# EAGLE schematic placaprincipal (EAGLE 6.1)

## Sheet 1 of 3: Diagrama Esquematico de Microcontrolador ATMEGA32U4: El siguiente esquema muestra las distribucion de los pines del microcontrolador junto con el Puerto USB que contiene este, ademas se tiene que tomar en cuenta que el se tiene 2 fuentes distintas la cual es una diferente del otra ya que una es VCC1 alimentacion del todo el circuito y VCC2 que es la alimentacion que viene del puerto USB
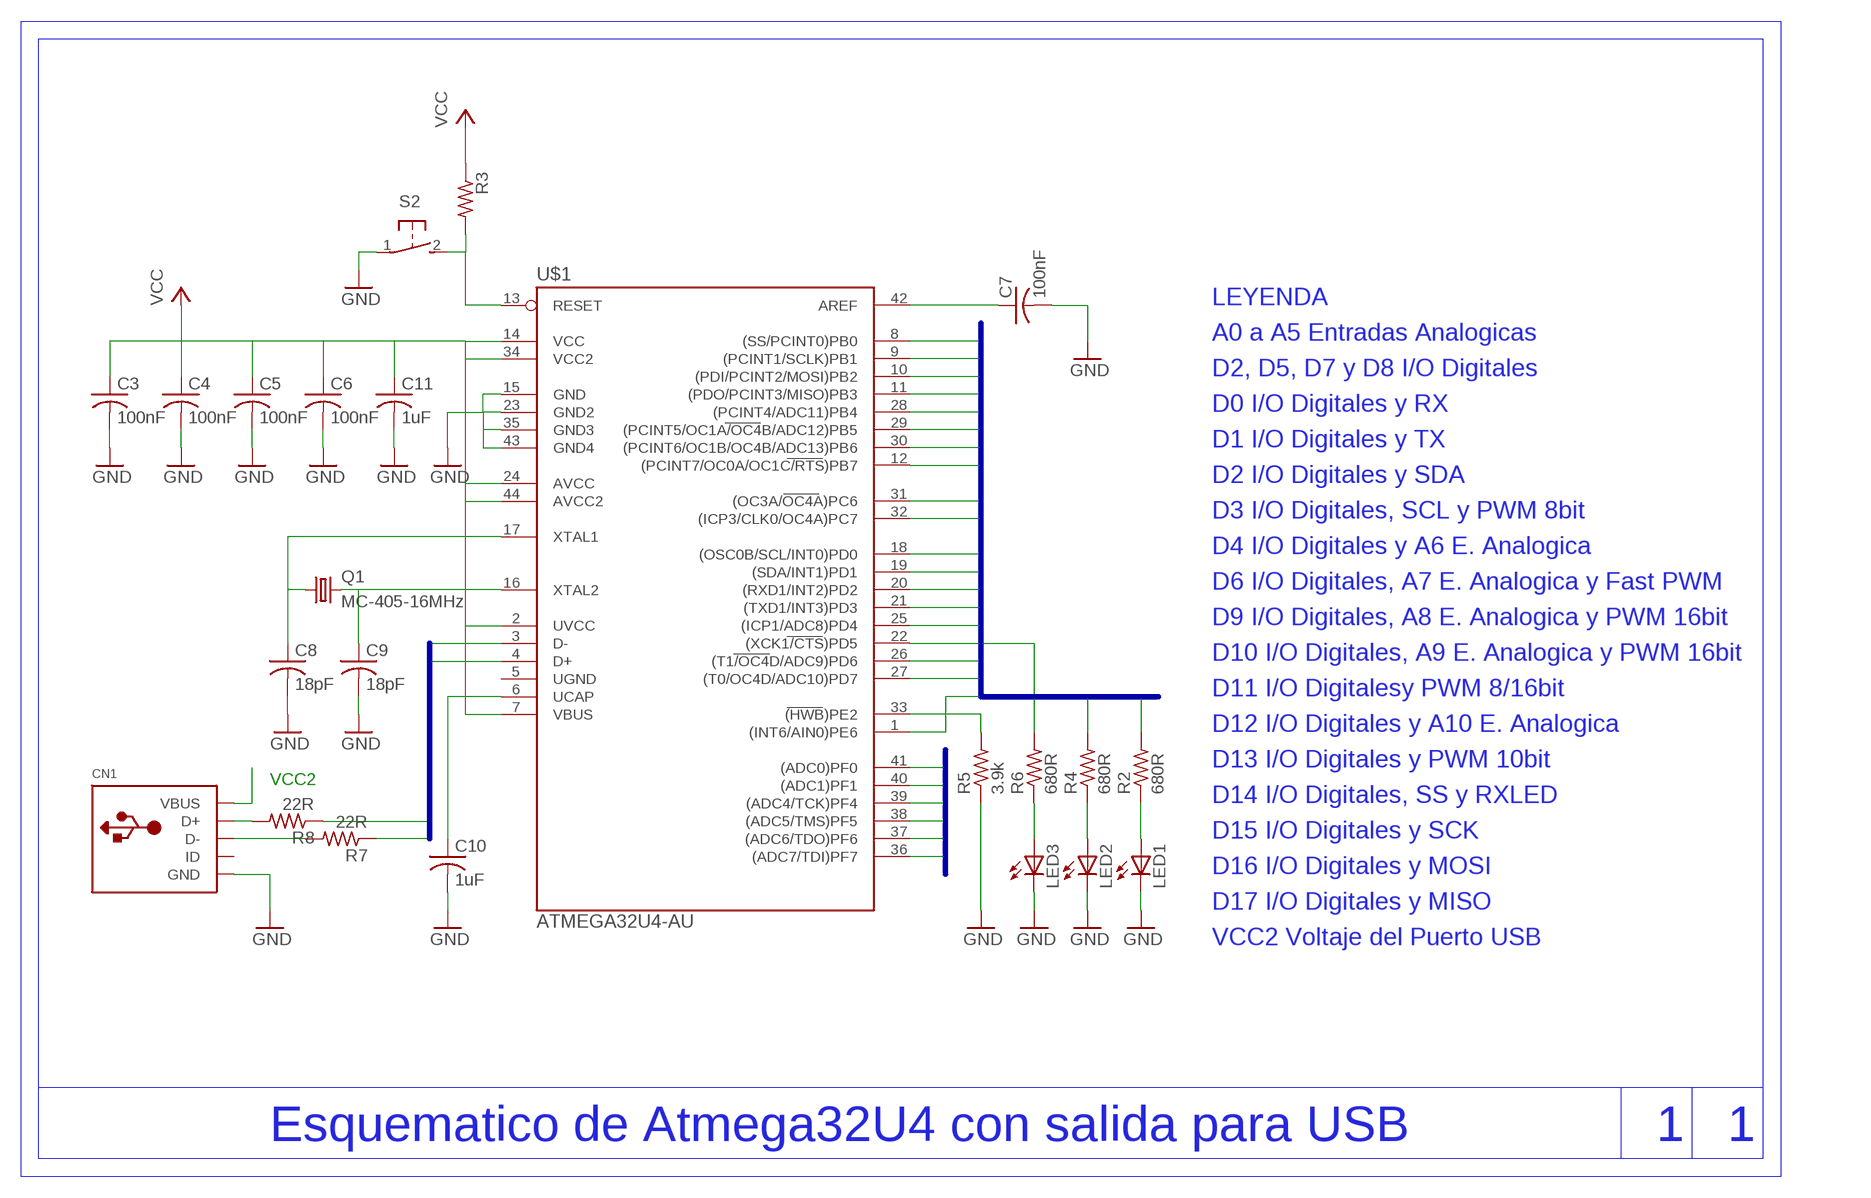
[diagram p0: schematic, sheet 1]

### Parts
C3  100nF  C-USC1206  [C1206]
C4  100nF  C-USC1206  [C1206]
C5  100nF  C-USC1206  [C1206]
C6  100nF  C-USC1206  [C1206]
C7  100nF  C-USC1206  [C1206]
C8  18pF  C-USC1206  [C1206]
C9  18pF  C-USC1206  [C1206]
C10  1uF  C-USC1206  [C1206]
C11  1uF  C-USC1206  [C1206]
CN1  USBMINIB  [USB-MINIB]
LED1  LEDSMT1206  [1206]
LED2  LEDSMT1206  [1206]
LED3  LEDSMT1206  [1206]
Q1  MC-405-16MHz  MC-405  [MC-405]
R2  680R  R-US_R1206  [R1206]
R3  R-US_R1206  [R1206]
R4  680R  R-US_R1206  [R1206]
R5  3.9k  R-US_R1206  [R1206]
R6  680R  R-US_R1206  [R1206]
R7  22R  R-US_R1206  [R1206]
R8  22R  R-US_R1206  [R1206]
S2  31-XX  [B3F-31XX]
U$1  ATMEGA32U4-AU  [TQFP44]

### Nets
A0: U$1.36((ADC7/TDI)PF7)
A1: U$1.37((ADC6/TDO)PF6)
A2: U$1.38((ADC5/TMS)PF5)
A3: U$1.39((ADC4/TCK)PF4)
A4: U$1.40((ADC1)PF1)
A5: U$1.41((ADC0)PF0)
D0: U$1.20((RXD1/INT2)PD2)
D1: U$1.21((TXD1/INT3)PD3)
D2: U$1.19((SDA/INT1)PD1) ; also sheet 2
D3: U$1.18((OSC0B/SCL/INT0)PD0) ; also sheet 2
D4: U$1.25((ICP1/ADC8)PD4)
D5: U$1.31((OC3A/OC4A)PC6)
D6: U$1.27((T0/OC4D/ADC10)PD7)
D7: U$1.1((INT6/AIN0)PE6)
D8: U$1.28((PCINT4/ADC11)PB4) ; also sheet 2
D9: U$1.29((PCINT5/OC1A/OC4B/ADC12)PB5)
D10: U$1.30((PCINT6/OC1B/OC4B/ADC13)PB6) ; also sheet 2
D11: U$1.12((PCINT7/OC0A/OC1C/RTS)PB7) ; also sheet 2
D12: U$1.26((T1/OC4D/ADC9)PD6) ; also sheet 2
D13: R4.2 U$1.32((ICP3/CLK0/OC4A)PC7) ; also sheet 2
D14: R2.2 U$1.8((SS/PCINT0)PB0)
D15: U$1.9((PCINT1/SCLK)PB1) ; also sheet 2
D16: U$1.10((PDI/PCINT2/MOSI)PB2) ; also sheet 2
D17: U$1.11((PDO/PCINT3/MISO)PB3) ; also sheet 2
DATA0: R7.1 U$1.3(D-)
DATA1: R8.1 U$1.4(D+)
GND: C3.2 C4.2 C5.2 C6.2 C7.2 C8.2 C9.2 C10.2 C11.2 CN1.GND LED1.C LED2.C LED3.C R5.1 S2.1(P) U$1.15(GND) U$1.23(GND2) U$1.35(GND3) U$1.43(GND4) ; also sheet 2,3
N$1: R5.2 U$1.33((HWB)PE2)
N$4: C10.1 U$1.6(UCAP)
N$5: C9.1 Q1.2 U$1.16(XTAL2)
N$6: C7.1 U$1.42(AREF)
N$7: C8.1 Q1.1 U$1.17(XTAL1)
N$9: R6.2 U$1.22((XCK1/CTS)PD5)
N$10: CN1.D- R7.2
N$11: R3.2 S2.2(S) U$1.13(RESET)
N$12: CN1.D+ R8.2
N$13: LED3.A R6.1
N$16: LED1.A R2.1
N$17: LED2.A R4.1
VCC: C3.1 C4.1 C5.1 C6.1 C11.1 R3.1 U$1.2(UVCC) U$1.7(VBUS) U$1.14(VCC) U$1.24(AVCC) U$1.34(VCC2) U$1.44(AVCC2) ; also sheet 2,3
VCC2: CN1.VBUS ; also sheet 3
Unconnected: CN1.ID U$1.5(UGND)

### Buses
A[0..5]
D[0..17]
DATA[0..1]

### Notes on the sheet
- LEYENDA
- A0 a A5 Entradas Analogicas
- D2, D5, D7 y D8 I/O Digitales
- D0 I/O Digitales y RX
- D1 I/O Digitales y TX
- D2 I/O Digitales y SDA
- D3 I/O Digitales, SCL y PWM 8bit
- D4 I/O Digitales y A6 E. Analogica
- D6 I/O Digitales, A7 E. Analogica y Fast PWM
- D9 I/O Digitales, A8 E. Analogica y PWM 16bit
- D10 I/O Digitales, A9 E. Analogica y PWM 16bit
- D11 I/O Digitalesy PWM 8/16bit
- D12 I/O Digitales y A10 E. Analogica
- D13 I/O Digitales y PWM 10bit
- VCC2
- D14 I/O Digitales, SS y RXLED
- D15 I/O Digitales y SCK
- D16 I/O Digitales y MOSI
- D17 I/O Digitales y MISO
- VCC2 Voltaje del Puerto USB
- Esquematico de Atmega32U4 con salida para USB | 1 | 1

## Sheet 2 of 3: Esquematicos de EPROM, RTC, SD y SIM908: Los cuales van unidos a la placa principal del microcontrolador mediante buses que nos permiten unir pines, en nuestro caso nos permite unir a las I/O digitales.
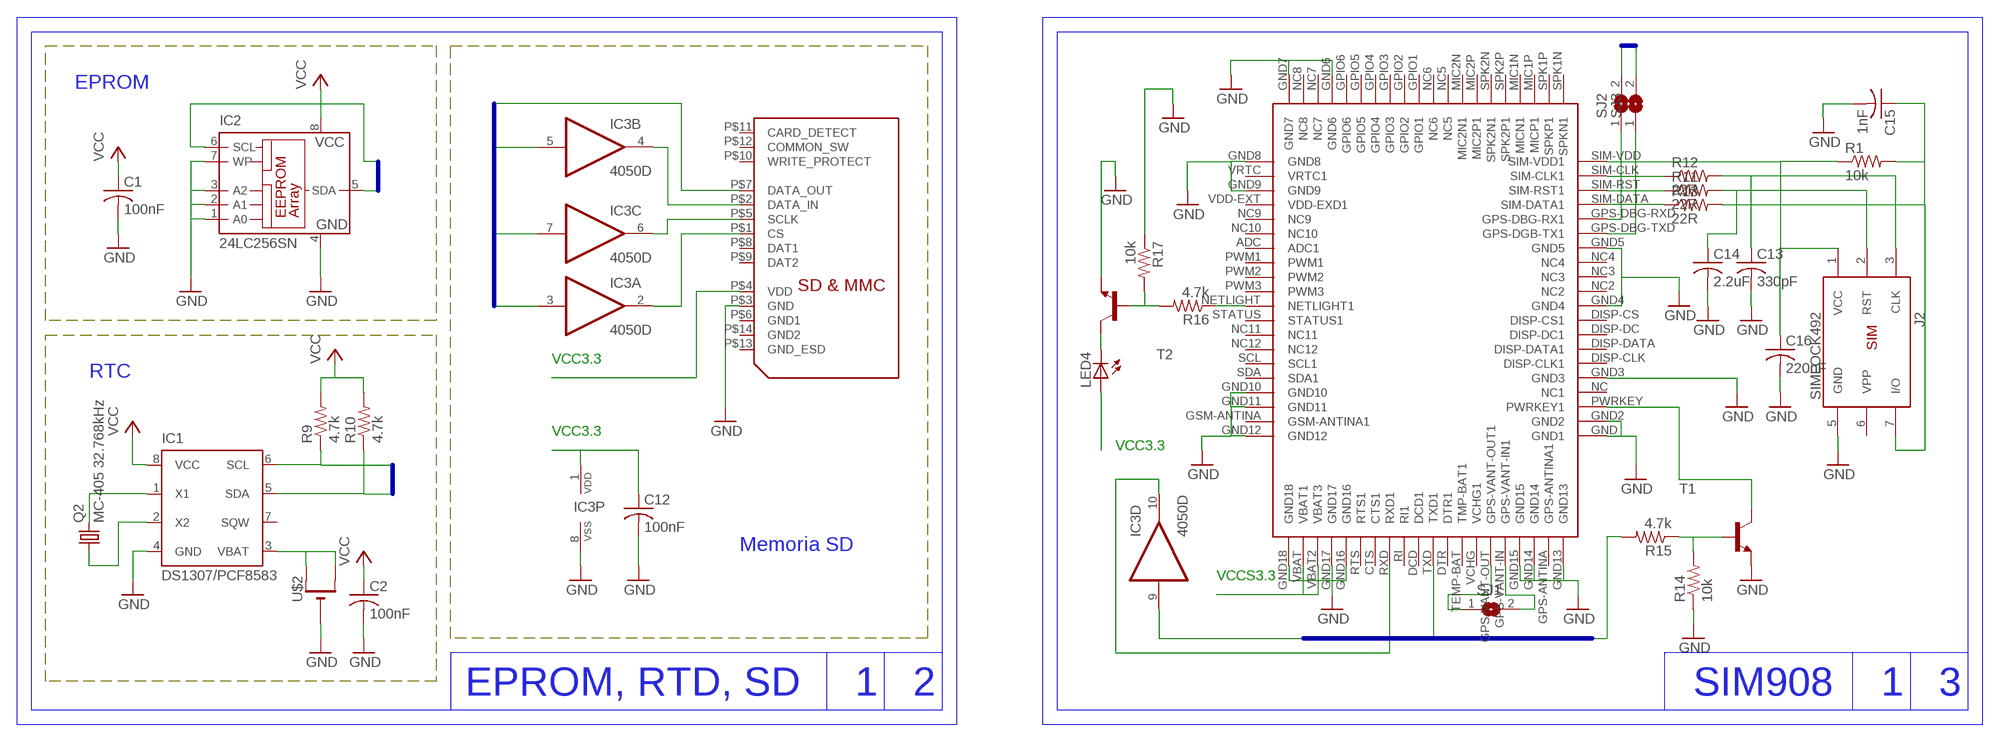
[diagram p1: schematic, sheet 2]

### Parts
C1  100nF  C-USC1206  [C1206]
C2  100nF  C-USC1206  [C1206]
C12  100nF  C-USC1206  [C1206]
C13  330pF  C-USC1206  [C1206]
C14  2.2uF  C-USC1206  [C1206]
C15  1nF  C-USC1206  [C1206]
C16  220nF  C-USC1206  [C1206]
IC1  DS1307/PCF8583  [SO8-7_5+SOIC8]
IC2  24LC256SN  [SO-08]
IC3  4050D  [SO16]
J2  SIMLOCK492  [5002]
LED4  LEDSMT1206  [1206]
Q2  MC-405 32.768kHz  MC-405  [MC-405]
R1  10k  R-US_R1206  [R1206]
R9  4.7k  R-US_R1206  [R1206]
R10  4.7k  R-US_R1206  [R1206]
R11  22R  R-US_R1206  [R1206]
R12  22R  R-US_R1206  [R1206]
R13  22R  R-US_R1206  [R1206]
R14  10k  R-US_R1206  [R1206]
R15  4.7k  R-US_R1206  [R1206]
R16  4.7k  R-US_R1206  [R1206]
R17  10k  R-US_R1206  [R1206]
SD1  FPS009-2405-0  [FPS009-2405]
SJ1  SJ  [SJ]
SJ2  SJ  [SJ]
SJ3  SJ  [SJ]
T1  BC817-16-NPN-SOT23-BEC  [SOT23-BEC]
T2  BC817-16-NPN-SOT23-BEC  [SOT23-BEC]
U$2  CR1220SMT  [CR1220-SMD]
U$4  SIM908  [SIM908]

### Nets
D2: IC1.5(SDA) IC2.5(SDA) R10.1 ; also sheet 1
D3: IC1.6(SCL) IC2.6(SCL) R9.1 ; also sheet 1
D8: R15.2 ; also sheet 1
D10: SJ2.2 ; also sheet 1
D11: IC3.3(A:I) SJ3.2 ; also sheet 1
D12: IC3.9(D:I) ; also sheet 1
D13: U$4.TXD(TXD1) ; also sheet 1
D15: IC3.7(C:I) ; also sheet 1
D16: IC3.5(B:I) ; also sheet 1
D17: SD1.P$7(DATA_OUT) ; also sheet 1
GND: C1.2 C2.2 C12.2 C13.2 C14.2 C15.2 C16.2 IC1.4(GND) IC2.1(A0) IC2.2(A1) IC2.3(A2) IC2.4(GND) IC2.7(WP) IC3.8(P:VSS) J2.5(GND) R14.1 R17.1 SD1.P$3(GND) T1.E T2.E U$2.- U$4.GND2 U$4.GND3 U$4.GND4 U$4.GND5 U$4.GND6 U$4.GND7 U$4.GND8 U$4.GND9 U$4.GND10 U$4.GND11 U$4.GND12 U$4.GND13 U$4.GND14 U$4.GND15 U$4.GND16 U$4.GND17 U$4.GND18 U$4.GND(GND1) ; also sheet 1,3
N$2: IC1.3(VBAT) U$2.+$1(+) U$2.+$2(+1)
N$3: IC1.1(X1) Q2.2
N$8: IC1.2(X2) Q2.1
N$14: IC3.2(A:O) SD1.P$1(CS)
N$15: IC3.4(B:O) SD1.P$2(DATA_IN)
N$18: IC3.6(C:O) SD1.P$5(SCLK)
N$19: C14.1 J2.2(RST) R11.2
N$20: C13.1 J2.3(CLK) R12.2
N$21: C15.1 J2.7(I/O) R1.2 R13.2
N$22: C16.1 J2.1(VCC) R1.1 U$4.SIM-VDD(SIM-VDD1)
N$23: R13.1 U$4.SIM-DATA(SIM-DATA1)
N$24: R12.1 U$4.SIM-CLK(SIM-CLK1)
N$25: R11.1 U$4.SIM-RST(SIM-RST1)
N$28: IC3.10(D:O) U$4.RXD(RXD1)
N$29: SJ2.1 U$4.GPS-DBG-RXD(GPS-DBG-RX1)
N$30: SJ3.1 U$4.GPS-DBG-TXD(GPS-DGB-TX1)
N$31: T1.C U$4.PWRKEY(PWRKEY1)
N$32: R14.2 R15.1 T1.B
N$33: R16.1 U$4.NETLIGHT(NETLIGHT1)
N$34: LED4.C T2.C
N$35: R16.2 R17.2 T2.B
N$38: SJ1.2 U$4.GPS-VANT-IN(GPS-VANT-IN1)
N$39: SJ1.1 U$4.GPS-VANT-OUT(GPS-VANT-OUT1)
VCC: C1.1 C2.1 IC1.8(VCC) IC2.8(VCC) R9.2 R10.2 ; also sheet 1,3
VCC3.3: C12.1 IC3.1(P:VDD) LED4.A SD1.P$4(VDD) U$4.VBAT2(VBAT3) U$4.VBAT(VBAT1) ; also sheet 3
Unconnected: IC1.7(SQW) IC3.11(E:I) IC3.12(E:O) IC3.14(F:I) IC3.15(F:O) J2.6(VPP) SD1.P$6(GND1) SD1.P$8(DAT1) SD1.P$9(DAT2) SD1.P$10(WRITE_PROTECT) SD1.P$11(CARD_DETECT) SD1.P$12(COMMON_SW) SD1.P$13(GND_ESD) SD1.P$14(GND2) U$4.ADC(ADC1) U$4.CTS(CTS1) U$4.DCD(DCD1) U$4.DISP-CLK(DISP-CLK1) U$4.DISP-CS(DISP-CS1) U$4.DISP-DATA(DISP-DATA1) U$4.DISP-DC(DISP-DC1) U$4.DTR(DTR1) U$4.GPIO1 U$4.GPIO2 U$4.GPIO3 U$4.GPIO4 U$4.GPIO5 U$4.GPIO6 U$4.GPS-ANTINA(GPS-ANTINA1) U$4.GSM-ANTINA(GSM-ANTINA1) U$4.MIC1N(MICN1) U$4.MIC1P(MICP1) U$4.MIC2N(MIC2N1) U$4.MIC2P(MIC2P1) U$4.NC2 U$4.NC3 U$4.NC4 U$4.NC5 U$4.NC6 U$4.NC7 U$4.NC8 U$4.NC9 U$4.NC10 U$4.NC11 U$4.NC12 U$4.NC(NC1) U$4.PWM1 U$4.PWM2 U$4.PWM3 U$4.RI(RI1) U$4.RTS(RTS1) U$4.SCL(SCL1) U$4.SDA(SDA1) U$4.SPK1N(SPKN1) U$4.SPK1P(SPKP1) U$4.SPK2N(SPK2N1) U$4.SPK2P(SPK2P1) U$4.STATUS(STATUS1) U$4.TEMP-BAT(TMP-BAT1) U$4.VCHG(VCHG1) U$4.VDD-EXT(VDD-EXD1) U$4.VRTC(VRTC1)

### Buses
D[0..17]

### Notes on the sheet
- EPROM
- VCC3.3
- RTC
- VCC3.3
- VCC3.3
- Memoria SD
- VCCS3.3
- EPROM, RTD, SD | 1 | 2 | SIM908 | 1 | 3

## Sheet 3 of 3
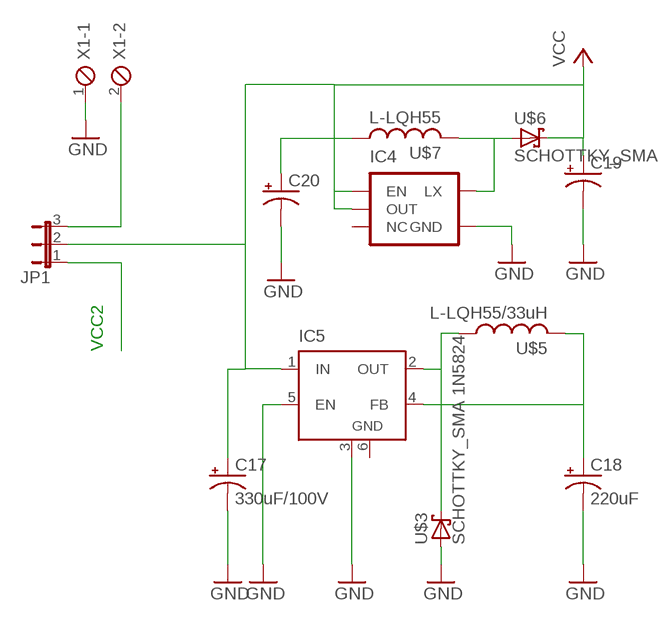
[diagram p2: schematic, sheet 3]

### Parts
C17  330uF/100V  CPOL-USD/7343-31W  [D/7343-31W]
C18  220uF  CPOL-USD/7343-31W  [D/7343-31W]
C19  CPOL-USD/7343-31W  [D/7343-31W]
C20  CPOL-USD/7343-31W  [D/7343-31W]
IC4  V_REG_NCP1400SOT23-5  [SOT23-5]
IC5  LM2596S  [TO263-5]
JP1  JP2E  [JP2]
U$3  SCHOTTKY_SMA 1N5824  SCHOTTKY_SMA  [SMA]
U$5  L-LQH55/33uH  L-LQH55  [LQH55]
U$6  SCHOTTKY_SMA  [SMA]
U$7  L-LQH55  [LQH55]
X1  MPT2  [2POL254]

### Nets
GND: C17.- C18.- C19.- C20.- IC4.4(GND) IC5.3(GND) IC5.5(EN) U$3.A X1.1 ; also sheet 1,2
N$26: JP1.3 X1.2
N$27: IC5.2(OUT) U$3.K(C) U$5.1
N$36: IC4.5(LX) U$6.A U$7.2
N$40: C20.+ U$7.1
VCC: C17.+ C19.+ IC4.1(EN) IC4.2(OUT) IC5.1(IN) JP1.2 U$6.K(C) ; also sheet 1,2
VCC2: JP1.1 ; also sheet 1
VCC3.3: C18.+ IC5.4(FB) U$5.2 ; also sheet 2
Unconnected: IC4.3(NC)

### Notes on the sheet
- VCC2

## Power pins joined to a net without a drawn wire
GND: IC5.6(GND)

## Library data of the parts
C1 C2 C12-C16 = rcl:C-US: CAPACITOR, American symbol
C3-C11 = adafruit:C-US: CAPACITOR, American symbol
C17-C20 = rcl:CPOL-US: POLARIZED CAPACITOR, American symbol
CN1 = adafruit:USB: USB Connectors USBMINIB - Surface Mount Female Mini-B USB Connector 4UConnector: 06564 By microbuilder.eu Thru-hole RA Female Mini-B USB Connector 4UConnector: 18732 By ladyada.net
IC1 = ds1307_pcf8583:DS1307: I2C-Bus CLOCK/CALENDAR
IC2 = microchip:24*: Serial EEPROM I2C; MF: MICROCHIP; MPN: 24LC256-I/SN; OC_FARNELL: 9757996; OC_NEWARK: 27C9144
IC3 = 40xx:4050: Hex non-inverting BUFFER
IC4 = SparkFun-PowerIC:V_REG_NCP1400: Switching step-up voltage regulator NCP1400 switiching regulator takes single cell AA and outputs 100mA at 3.3V or 5V with minimal number of external components.
IC5 = linear:LM2596S: STEP-DOWN VOLTAGE REGULATOR
J2 = amphenol-simlock:SIMLOCK492
JP1 = jumper:JP2E: JUMPER
LED1-LED3 = adafruit:LED: LED
LED4 = led:LED: LED
Q1 Q2 = crystal:MC-405: kHz RANGE CRYSTAL UNIT SMD; OC_FARNELL: unknown; OC_NEWARK: unknown
R1 R9-R17 = rcl:R-US_: RESISTOR, American symbol
R2-R8 = adafruit:R-US_: RESISTOR, American symbol
S2 = switch-omron:31-XX: OMRON SWITCH; MPN: B3F-3100; OC_FARNELL: 959704; OC_NEWARK: 36M3582
SD1 = con-yamaichi2:FPS009-2405-0
SJ1-SJ3 = jumper:SJ: SMD solder JUMPER
T1 T2 = transistor:*-NPN-: NPN Transistror BF959 corrected 2008.03.06
U$1 = mega32U4:ATMEGA32U4-AU
U$2 = adafruit:CR1220: CR1216/CR1220/CR1225 12mm 3V lithium coin cell Great for battery packup. Both SMT and THM holders. Note the THM package has the ground pads on both sides of the PCB so that the masks are the same - this reduces the cost
U$3 U$6 = casovac:SCHOTTKY_SMA
U$4 = sim908_-made_by_hardik:SIM908
U$5 U$7 = adafruit:L
X1 = con-phoenix-254:MPT2: PHOENIX CONNECTOR; OC_FARNELL: unknown; OC_NEWARK: unknown

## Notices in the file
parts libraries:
SparkFun-PowerIC: Licensing: Creative Commons ShareAlike 4.0 International - https://creativecommons.org/licenses/by-sa/4.0
